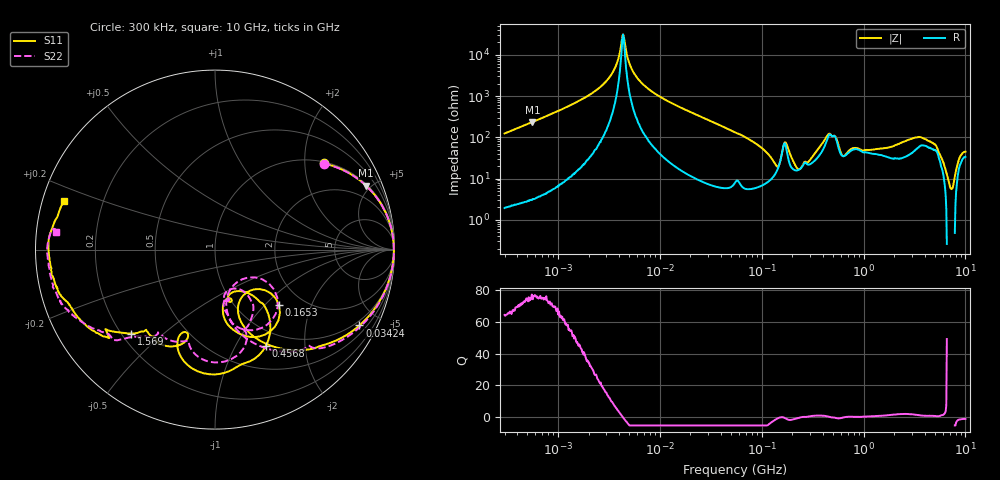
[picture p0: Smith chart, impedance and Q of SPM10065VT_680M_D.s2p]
! S-Parameter Data Generated by TDK Corporation
! Copyright(C) 2020 TDK Corporation.
! All Rights Reserved.
! TDK P/N: SPM10065VT-680M-D (Inductor)
! Property: L=68uH at 100kHz
! Size(LxWxT): 10.5x10x6.5mm
! Model Type: s2p (Touchstone File Format Version 1.0)
! Frequency: DC=Yes Start=0.3MHz Stop=10000MHz 802points Log-sweep
! Model Generated on Aug. 18, 2020
! Port Assignments:
!  1 ---@@@--- 2
! Applicable Conditions:
!  Temperature = 25 degC
!  DC Bias Current = 0 A
!  Small Signal Operation
! Terms and conditions regarding TDK Simulation Models
! (1)This simulation model is being provided solely for informational purposes. Please refer to the specifications of the products in terms of detailed characteristics of such products.
! (2)In no event shall TDK Corporation of any of its subsidiaries be liable for any loss or damage arising, directly or indirectly,
!  From any information contained in this simulation model, including, but not limited to loss or damages arising from any inaccuracies, omissions or errors in connection with such information.
! (3)Any and all copyrights on this simulation model are owned by TDK Corporation.
!  Duplication or redistribution of this simulation model without prior written permission from TDK Corporation is prohibited.
! (4)This simulation model is subject to any modification or change without any prior notice.
! (5)Neither TDK Corporation nor any of its subsidiaries shall make any warranty, express or implied,
!  Including but not limited to the correctness, implied warranties of merchantability and fitness for a particular purpose with respect to this simulation models.
! (6)The use of this simulation model shall be deemed to have consented to the terms and conditions hereof.
# Hz S MA R 50
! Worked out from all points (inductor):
!   801 points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, 300 kHz to 10 GHz, reference 50 ohm
!   read as one part in series: L = 65.3 uH near 318.3 kHz
!   highest Q = 75.3 at 561.4 kHz (marker M1), where L = 66.3 uH
!   self-resonance near 4.363 MHz
!   S11 on the Smith chart (normalised r, x): 300 kHz: 1.04, +2.48; 34.24 MHz: 0.80, -3.90; 165.3 MHz: 1.52, -1.22; 456.8 MHz: 0.79, -1.34; 1.569 GHz: 0.24, -0.39; 10 GHz: 0.06, +0.16
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300000  0.7727 38.5  0.6238 -50.7  0.6232 -50.7  0.7719 38.4
561390  0.914 23.0  0.3908 -66.3  0.3908 -66.3  0.9142 22.9
1713600  0.9893 6.7  0.1195 -82.0  0.1195 -82.0  0.9897 6.6
3240674  0.9961 1.5  0.03388 -83.7  0.03381 -83.6  0.9965 1.4
4363314  0.9964 -0.6  0.003207 -2.0  0.003061 -2.0  0.9968 -0.8
5612817  0.9959 -2.4  0.02838 80.8  0.02839 80.8  0.9963 -2.6
9671944  0.9908 -6.9  0.09714 80.5  0.09713 80.5  0.9911 -7.3
3.424315e7  0.909 -27.7  0.3915 59.9  0.3914 59.9  0.9084 -29.3
5.477226e7  0.8017 -41.7  0.5621 43.6  0.5619 43.6  0.7748 -45.0
1.258969e8  0.4081 -70.4  0.8337 3.4  0.8335 3.4  0.3902 -78.2
1.495617e8  0.297 -53.6  0.7946 -12.7  0.7944 -12.7  0.2237 -62.2
1.653189e8  0.4725 -41.0  0.5765 -16.4  0.5764 -16.4  0.3989 -34.1
1.855783e8  0.5135 -70.1  0.6909 -1.0  0.6908 -1.0  0.484 -68.0
3.126428e8  0.258 -69.1  0.766 -39.7  0.7658 -39.7  0.2383 -71.5
3.7738e8  0.3292 -50.8  0.6442 -58.4  0.6442 -58.4  0.3145 -54.4
4.568044e8  0.6059 -62.0  0.3592 -61.9  0.3591 -61.9  0.457 -65.6
5.285151e8  0.6931 -87.7  0.3523 -43.7  0.3523 -43.7  0.5744 -74.1
6.076905e8  0.5923 -110.4  0.5154 -44.3  0.5153 -44.3  0.602 -99.3
1.569319e9  0.6612 -135.0  0.2771 -131.1  0.2771 -131.1  0.6578 -132.5
1.767019e9  0.7031 -139.0  0.2256 -146.5  0.2256 -146.5  0.6975 -135.0
4.924213e9  0.9126 -168.9  0.02009 -168.3  0.02006 -168.3  0.916 -164.3
1e10  0.8826 162.1  0.02664 141.5  0.02662 141.5  0.8919 173.7
